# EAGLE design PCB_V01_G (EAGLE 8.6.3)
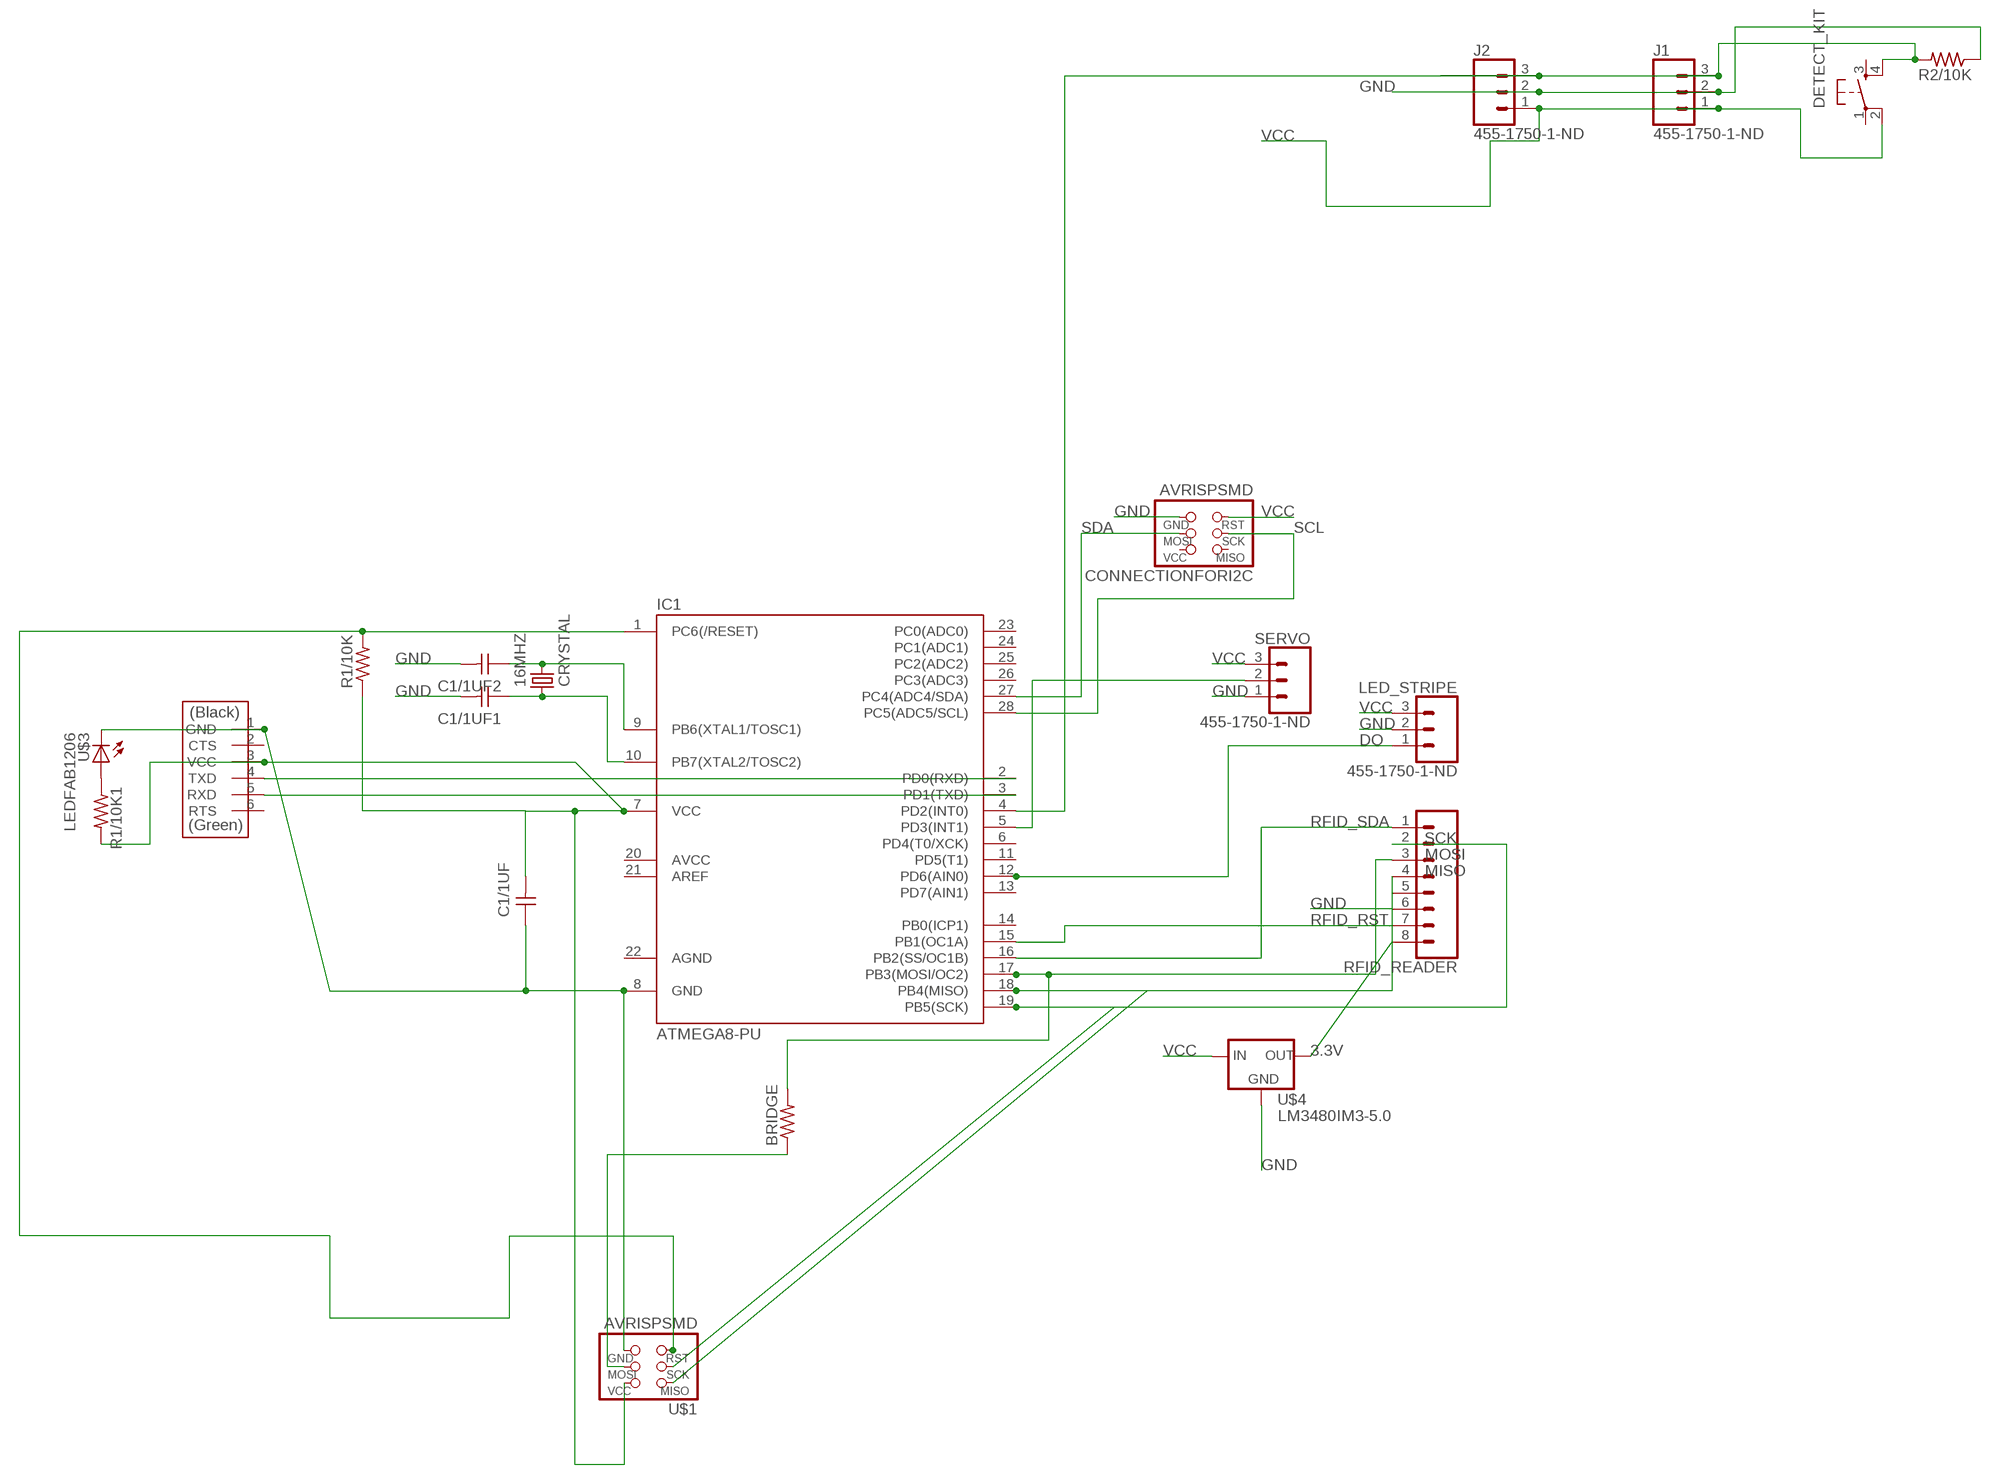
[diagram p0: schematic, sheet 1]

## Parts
16MHZ  CRYSTAL  [2-SMD-5X3MM]
BRIDGE  RES-US1206FAB  [R1206FAB]
C1/1UF  CAP-UNPOLARIZEDFAB  [C1206FAB]
C1/1UF1  CAP-UNPOLARIZEDFAB  [C1206FAB]
C1/1UF2  CAP-UNPOLARIZEDFAB  [C1206FAB]
CONNECTIONFORI2C  AVRISPSMD  [2X03SMD]
DETECT_KIT  6MM_SWITCH6MM_SWITCH  [6MM_SWITCH]
IC1  ATMEGA8-PU  [DIL28-3]
J1  455-1750-1-ND  CONN_03  [1X03]
J2  455-1750-1-ND  CONN_03  [1X03]
LED_STRIPE  455-1750-1-ND  CONN_03  [1X03]
R1/10K  RES-US1206FAB  [R1206FAB]
R1/10K1  RES-US1206FAB  [R1206FAB]
R2/10K  RES-US1206FAB  [R1206FAB]
RFID_READER  CONN_08"  [1X08]
SERVO  455-1750-1-ND  CONN_03  [1X03]
U$1  AVRISPSMD  [2X03SMD]
U$2  FTDI-SMD-HEADER  [1X06SMD]
U$3  LEDFAB1206  [LED1206FAB]
U$4  LM3480IM3-5.0  [SOT23]

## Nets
3.3V: RFID_READER.8 U$4.1(OUT)
DO: IC1.12(PD6(AIN0)) LED_STRIPE.1
GND: C1/1UF1.2 C1/1UF2.2 C1/1UF.1 CONNECTIONFORI2C.6(GND) IC1.8(GND) J1.2 J2.2 LED_STRIPE.2 R2/10K.1 RFID_READER.6 SERVO.1 U$1.6(GND) U$2.1(GND) U$3.2(C) U$4.3(GND)
MISO: IC1.18(PB4(MISO)) RFID_READER.4 U$1.1(MISO)
MOSI: BRIDGE.2 IC1.17(PB3(MOSI/OC2)) RFID_READER.3
N$1: BRIDGE.1 U$1.4(MOSI)
N$2: R1/10K1.1 U$3.1(A)
N$3: 16MHZ.P$2 C1/1UF2.1 IC1.9(PB6(XTAL1/TOSC1))
N$4: IC1.5(PD3(INT1)) SERVO.2
N$5: 16MHZ.P$1 C1/1UF1.1 IC1.10(PB7(XTAL2/TOSC2))
N$8: IC1.3(PD1(TXD)) U$2.5(RXD)
N$9: IC1.2(PD0(RXD)) U$2.4(TXD)
N$10: DETECT_KIT.4(S1) IC1.4(PD2(INT0)) J1.3 J2.3 R2/10K.2
N$14: IC1.1(PC6(/RESET)) R1/10K.2 U$1.5(RST)
RFID_RST: IC1.15(PB1(OC1A)) RFID_READER.7
RFID_SDA: IC1.16(PB2(SS/OC1B)) RFID_READER.1
SCK: IC1.19(PB5(SCK)) RFID_READER.2 U$1.3(SCK)
SCL: CONNECTIONFORI2C.3(SCK) IC1.28(PC5(ADC5/SCL))
SDA: CONNECTIONFORI2C.4(MOSI) IC1.27(PC4(ADC4/SDA))
VCC: C1/1UF.2 CONNECTIONFORI2C.5(RST) DETECT_KIT.2(P1) IC1.7(VCC) J1.1 J2.1 LED_STRIPE.3 R1/10K1.2 R1/10K.1 SERVO.3 U$1.2(VCC) U$2.3(VCC) U$4.2(IN)
Unconnected: CONNECTIONFORI2C.1(MISO) CONNECTIONFORI2C.2(VCC) DETECT_KIT.1(P) DETECT_KIT.3(S) IC1.6(PD4(T0/XCK)) IC1.11(PD5(T1)) IC1.13(PD7(AIN1)) IC1.14(PB0(ICP1)) IC1.20(AVCC) IC1.21(AREF) IC1.23(PC0(ADC0)) IC1.24(PC1(ADC1)) IC1.25(PC2(ADC2)) IC1.26(PC3(ADC3)) RFID_READER.5 U$2.2(CTS) U$2.6(RTS)

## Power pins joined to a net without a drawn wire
AGND: IC1.22(AGND)

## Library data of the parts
16MHZ = fab:CRYSTAL
BRIDGE R1/10K R1/10K1 R2/10K = fab:RES-US: Resistor (US Symbol)
C1/1UF C1/1UF1 C1/1UF2 = fab:CAP-UNPOLARIZED
CONNECTIONFORI2C U$1 = fab:AVRISP
DETECT_KIT = fab:6MM_SWITCH: OMRON SWITCH
IC1 = atmega8:ATMEGA8-PU
J1 J2 LED_STRIPE SERVO = SparkFun-Connectors:CONN_03: Multi connection point. Often used as Generic Header-pin footprint for 0.1 inch spaced/style header connections On any of the 0.1 inch spaced packages, you can populate with these: Break Away Headers - Straight (PRT-00116) Break Away Male Headers - Right Angle (PRT-00553) Female Headers (PRT-00115)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; PROD_ID: XXX-00000
RFID_READER = SparkFun-Connectors:CONN_08: Multi connection point. Often used as Generic Header-pin footprint for 0.1 inch spaced/style header connections On any of the 0.1 inch spaced packages, you can populate with these: Break Away Headers - Straight (PRT-00116) Break Away Male Headers - Right Angle (PRT-00553) Female Headers (PRT-00115)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; PROD_ID: CONN-08438
U$2 = fab:FTDI-SMD-HEADER
U$3 = fab:LED: LED
U$4 = national_gaui:LM3480

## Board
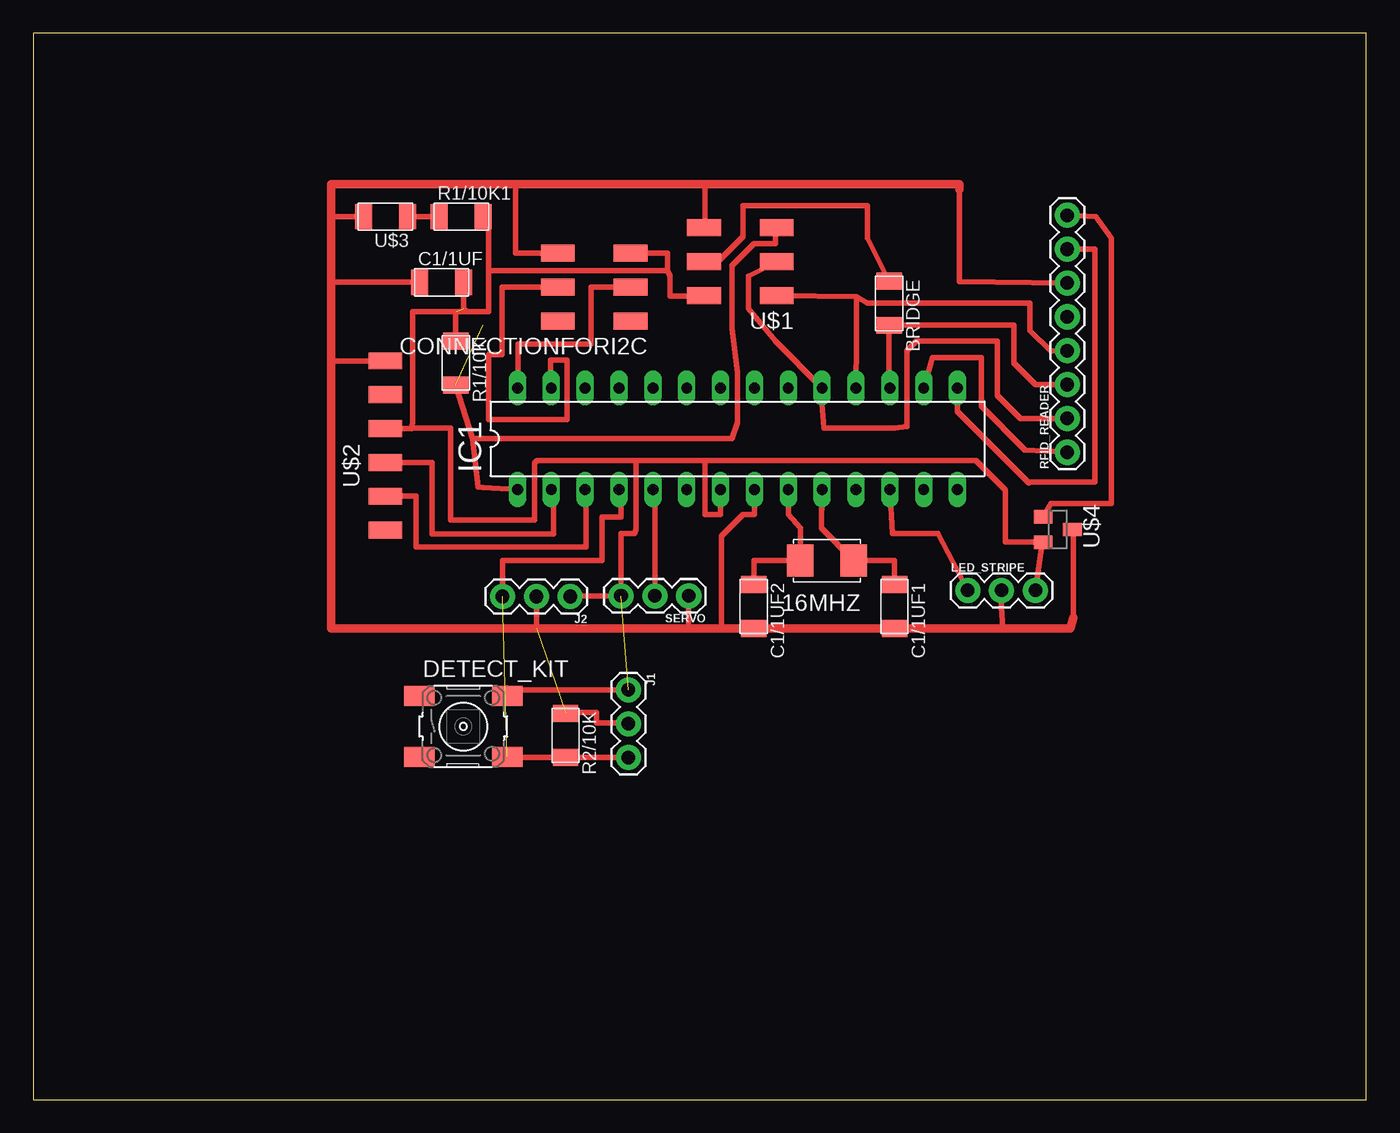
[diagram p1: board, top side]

Size 100 x 80 mm. Coordinates in mm from the lower left corner, seen from the top.
Outline: 0,0 100,0 100,80 0,80 0,0
Copper layers (1*16): Top 0.035mm / dielectric 1.5mm / Bottom 0.035mm
Design rules "default *": minimum track width 6mil, minimum drill 0.35mm, track to track 16mil, track to pad 16mil, pad to pad 16mil, via to via 16mil, smd to smd 16mil, copper to edge 40mil, drill to drill 6mil, minimum pad ring 10mil, minimum via ring 8mil, stop-mask expansion 4mil, vias tented up to drill 0mil, thermal gap 10mil

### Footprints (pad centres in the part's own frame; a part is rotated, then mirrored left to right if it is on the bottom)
2-SMD-5X3MM = smd 2 x 2.4: P$1 -2,0; P$2 2,0
R1206FAB = smd 1.27 x 1.905: 1 -1.651,0; 2 1.651,0
C1206FAB = smd 1.27 x 1.905: 1 -1.651,0; 2 1.651,0
2X03SMD = smd 2.54 x 1.27: 1 -2.54,2.54; 2 2.92,2.54; 3 -2.54,0; 4 2.92,0; 5 -2.54,-2.54; 6 2.92,-2.54
6MM_SWITCH = smd 2.286 x 1.524: 1 -3.302,2.286; 2 3.302,2.286; 3 -3.302,-2.286; 4 3.302,-2.286
DIL28-3 = drill 0.813 long: 1 -16.51,-3.81; 2 -13.97,-3.81; 3 -11.43,-3.81; 4 -8.89,-3.81; 5 -6.35,-3.81; 6 -3.81,-3.81; 7 -1.27,-3.81; 8 1.27,-3.81; 9 3.81,-3.81; 10 6.35,-3.81; 11 8.89,-3.81; 12 11.43,-3.81; 13 13.97,-3.81; 14 16.51,-3.81; 15 16.51,3.81; 16 13.97,3.81; 17 11.43,3.81; 18 8.89,3.81; 19 6.35,3.81; 20 3.81,3.81; 21 1.27,3.81; 22 -1.27,3.81; 23 -3.81,3.81; 24 -6.35,3.81; 25 -8.89,3.81; 26 -11.43,3.81; 27 -13.97,3.81; 28 -16.51,3.81
1X03 = drill 1.016 pad 1.88: 1 0,0; 2 2.54,0; 3 5.08,0
1X08 = drill 1.016 pad 1.88: 1 0,0; 2 2.54,0; 3 5.08,0; 4 7.62,0; 5 10.16,0; 6 12.7,0; 7 15.24,0; 8 17.78,0
1X06SMD = smd 2.54 x 1.27: 1 0,6.35; 2 0,3.81; 3 0,1.27; 4 0,-1.27; 5 0,-3.81; 6 0,-6.35
LED1206FAB = smd 1.27 x 1.905: 1 -1.651,0; 2 1.651,0
SOT23 = smd 1 x 1.4: 1 -0.95,-1.1; 2 0.95,-1.1; 3 0,1.1

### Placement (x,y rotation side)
16MHZ  59.54,40.44 180 top
BRIDGE  64.21,59.74 270 top
C1/1UF  30.63,61.32 0 top
C1/1UF1  64.62,36.98 270 top
C1/1UF2  54.05,36.98 270 top
CONNECTIONFORI2C  42.27,60.96 180 top
DETECT_KIT  32.26,27.99 0 top
IC1  52.83,49.58 0 top
J1  44.65,30.73 270 top
J2  40.28,37.74 180 top
LED_STRIPE  70.1,38.2 0 top
R1/10K  31.7,55.27 270 top
R1/10K1  32.11,66.24 0 top
R2/10K  39.93,27.33 270 top
RFID_READER  77.57,48.56 90 top
SERVO  49.17,37.8 180 top
U$1  53.24,62.86 180 top
U$2  26.42,49.07 0 top
U$3  26.42,66.24 180 top
U$4  76.86,42.77 270 top

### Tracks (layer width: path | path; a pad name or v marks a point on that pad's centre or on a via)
3.3V
  Top 0.406: 75.95,43.91 U$4.1 76.33,44.7 80.87,44.7 80.87,64.62 79.7,66.24 RFID_READER.8
DO
  Top 0.406: IC1.12 64.47,42.47 67.87,42.47 LED_STRIPE.1
GND  (1 unrouted)
  Top 0.406: U$1.6 50.39,65.48 50.39,68.68 | RFID_READER.6 69.49,61.37 69.49,68.68 | U$4.3 78.03,42.77 78.03,36.17 | 22.35,61.37 22.35,61.32 C1/1UF.1 | U$3.2 22.35,66.24 | LED_STRIPE.2 72.64,36.96 72.75,35.33 | 51.61,35.36 51.61,42.27 53.24,43.89 54.05,43.89 54.1,43.94 IC1.8 | U$2.1 22.35,55.42 22.35,55.27 | J2.2 37.74,35.36 37.59,35.36 | SERVO.1 49.17,35.36 | CONNECTIONFORI2C.6 36.17,63.5 36.17,68.68 | R2/10K.1 39.93,29.06 42.27,29.06 42.27,28.25 44.65,28.25 J1.2
  Top 0.635: 69.49,68.28 69.49,68.68 50.39,68.68 36.17,68.68 22.35,68.68 22.35,66.24 22.35,61.37 22.35,55.27 22.35,35.36 37.59,35.36 49.17,35.36 51.61,35.36 52.4,35.36 C1/1UF2.2 C1/1UF1.2 72.75,35.33 77.8,35.33 78.03,36.17
MISO
  Top 0.406: U$1.1 61.77,60.25 | 61.77,60.25 61.75,56.9 IC1.18 | RFID_READER.4 76.4,56.14 76.34,56.14 74.78,57.71 74.78,59.74 62.59,59.74 61.77,60.25
MOSI
  Top 0.406: IC1.17 64.35,53.39 64.21,53.52 BRIDGE.2 66.62,58.09 73.56,58.12 73.56,55.27 75.18,53.65 RFID_READER.3
N$1
  Top 0.406: U$1.4 51.44,62.94 53.24,64.74 53.24,67.06 62.59,67.06 62.59,64.64 BRIDGE.1
N$2
  Top 0.406: R1/10K1.1 U$3.1
N$3
  Top 0.406: IC1.9 56.64,43.89 57.54,42.88 16MHZ.P$2 54.05,40.44 C1/1UF2.1
N$4
  Top 0.406: SERVO.2 46.63,45.77 IC1.5
N$5
  Top 0.406: IC1.10 59.18,44.3 59.13,44.3 59.13,42.88 16MHZ.P$1 64.62,40.44 C1/1UF1.1
N$8
  Top 0.406: IC1.3 41.45,45.72 41.45,41.45 28.73,41.45 28.73,45.26 U$2.5
N$9
  Top 0.406: IC1.2 39.01,45.62 39.01,42.42 29.92,42.42 29.92,47.8 U$2.4
N$10  (1 unrouted)
  Top 0.406: J2.3 35.2,40.44 42.67,40.44 42.67,43.69 44.09,43.69 44.09,45.77 IC1.4 | DETECT_KIT.4 35.56,25.68 R2/10K.2 39.93,25.65 J1.3
N$14  (1 unrouted)
  Top 0.406: R1/10K.2 32.94,49.58 | 32.94,49.58 33.35,45.95 33.73,45.92 IC1.1 | U$1.5 55.68,65.3 55.68,64.21 54.05,64.21 52.43,62.59 52.43,57.83 52.83,54.58 52.83,50.8 52.43,49.58 32.94,49.58
RFID_RST
  Top 0.406: RFID_READER.7 79.65,63.8 79.65,46.33 74.78,46.33 74.7,46.25 69.34,51.61 IC1.15
RFID_SDA
  Top 0.406: RFID_READER.1 74.37,48.74 74.37,48.77 71.12,52.02 71.12,55.68 67.46,55.68 IC1.16
SCK
  Top 0.406: U$1.3 53.65,61.77 53.65,59.33 55.68,56.9 IC1.19 59.18,52.17 59.33,50.39 64.62,50.39 65.53,50.49 65.53,56.19 66.24,56.9 72.34,56.9 72.34,52.83 74.07,51.1 RFID_READER.2
SCL
  Top 0.406: IC1.28 36.37,53.39 36.37,56.69 41.86,56.69 41.86,60.96 CONNECTIONFORI2C.3
SDA
  Top 0.406: CONNECTIONFORI2C.4 35.15,60.96 35.15,55.88 34.14,55.88 34.14,51 40.03,51 40.03,55.47 38.81,55.47 38.81,53.39 IC1.27
VCC  (2 unrouted)
  Top 0.406: 29.67,59.13 28.45,59.13 28.45,50.8 28.4,50.34 | 29.67,59.13 31.7,59.13 | 31.7,59.13 34.14,59.13 34.14,62.18 | 28.4,50.34 U$2.3 | U$1.2 50.29,60.3 47.75,60.3 47.75,61.77 47.57,62.2 | 29.67,59.13 29.64,59.11 | 50.39,47.95 70.71,47.95 72.95,45.72 72.95,41.82 U$4.2 75.72,41.86 LED_STRIPE.3 | R1/10K.1 31.7,59.13 | C1/1UF.2 32.28,59.36 32.51,59.13 | R1/10K1.2 34.14,65.86 34.14,62.18 | IC1.7 51.56,43.89 50.39,43.89 50.39,47.95 | 50.39,47.95 45.31,47.95 | 45.31,47.95 37.8,47.95 37.59,47.75 37.59,43.48 31.29,43.48 31.29,50.39 28.4,50.39 28.4,50.34 | J2.1 40.28,37.8 SERVO.3 44.09,42.47 45.11,42.47 45.11,42.45 45.21,42.76 45.21,47.85 45.31,47.95 | 34.14,62.18 35.56,62.18 36.2,62.2 47.57,62.2 | CONNECTIONFORI2C.5 47.57,63.5 47.57,62.2 | J1.1 35.56,30.73 | 35.56,30.73 35.56,30.89 | 35.56,30.73 DETECT_KIT.2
